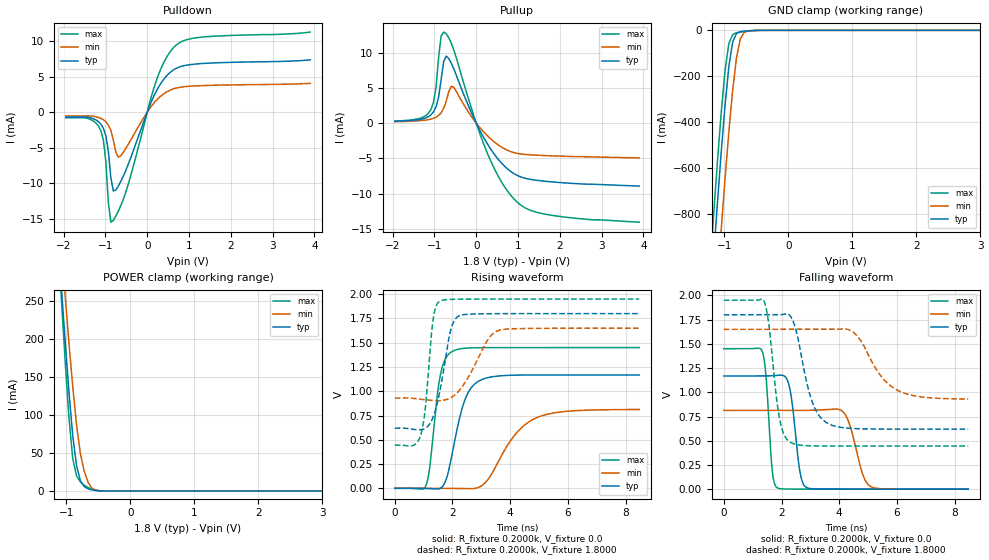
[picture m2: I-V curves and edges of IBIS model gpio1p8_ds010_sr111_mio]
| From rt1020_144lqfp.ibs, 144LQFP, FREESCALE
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[Model] gpio1p8_ds010_sr111_mio
|   Model gpio1p8_ds010_sr111_mio
| This model was characterised for following simulation conditions:
| External (pad) voltage:
|   - Typ: 1.8V,   - Min: 1.65V,   - Max: 1.95V
| Library cells for typ/min/max conditions are connected as defined below:
|  pad - External Pad
|  ipp_do - Core Input
|  ipp_obe - Output Buffer Enable
|  esd_boost - ovdd
|  ipp_dse0 - vssi
|  ipp_dse1 - vddi
|  ipp_dse2 - vssi
|  ipp_fsel0 - vddi
|  ipp_fsel1 - vddi
|  ipp_ina - ipp_ina
|  ipp_ind - ipp_ind
|  ipp_pwr_stable - vddi
|  ipp_sre - vddi
|  ovdd - ovdd
|  ovss - ovss
|  vddi - vddi
|  vssi - vssi
| All other pins connected to ground
Model_type I/O
Polarity   Non-Inverting
Enable   Active-High
Vinl =   0.5400V
Vinh =   1.2600V
Vmeas =  0.9000V
Cref =   0.0F
Rref =   0.2000k
Vref =   0.9000V
C_comp   1.2573pF   1.2208pF   1.3056pF
|C_comp_pullup   0.6440pF   0.6611pF   0.6285pF
|C_comp_pulldown   0.5474pF   0.5788pF   0.5258pF
[Model Spec]
| variable   typ   min   max
Vinh   1.2600V   1.1550V   1.3650V
Vinl   0.5400V   0.4950V   0.5850V
S_overshoot_high   1.8000V   1.6500V   1.9500V
S_overshoot_low   0.0V   0.0V   0.0V
Vmeas   0.9000V   0.8250V   0.9750V
Vref   0.9000V   0.8250V   0.9750V
Cref   0.0F   0.0F   0.0F
Rref   0.2000k   0.2000k   0.2000k
[Temperature Range]   25.0000   0.1050k   -20.0000
[Voltage Range]   1.8000V   1.6500V   1.9500V
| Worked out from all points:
|   slope of the pulldown table from 0 to 0.27 V, typ, clamps not added: 76.7 ohm
|   slope of the pullup table from 0 to 0.27 V, typ, clamps not added: 91 ohm
|   GND clamp passes 1 mA (typ) near -0.55 V on its own axis
|   POWER clamp passes 1 mA (typ) near -0.58 V on its own axis
|   rising waveform, R_fixture 0.2000k, V_fixture 0.0: 20-80 % time 556ps typ, 1.1ns min, 334ps max; typ from 0 V to 1.17 V
|   rising waveform, R_fixture 0.2000k, V_fixture 1.8000: 20-80 % time 431ps typ, 774ps min, 263ps max; typ from 0.619 V to 1.8 V
|   falling waveform, R_fixture 0.2000k, V_fixture 0.0: 20-80 % time 263ps typ, 424ps min, 185ps max; typ from 1.17 V to 0 V
|   falling waveform, R_fixture 0.2000k, V_fixture 1.8000: 20-80 % time 560ps typ, 950ps min, 339ps max; typ from 1.8 V to 0.619 V
[Pulldown]
|Voltage   I(typ)   I(min)   I(max)
-1.95V    -679uA     -527uA     -778uA
-1.41V    -700uA     -513uA     -902uA
-1.11V    -1.667mA   -870uA     -2.597mA
-990mV    -3.318mA   -1.338mA   -6.94mA
-930mV    -5.527mA   -1.788mA   -12.74mA
-870mV    -9.21mA    -2.57mA    -15.45mA
-810mV    -11.08mA   -3.94mA    -15.19mA
-750mV    -10.91mA   -5.632mA   -14.56mA
-630mV    -9.694mA   -6.09mA    -13.08mA
210mV     2.875mA    1.617mA    4.3mA
690mV     6.147mA    3.383mA    9.407mA
3.9V      7.35mA     4.05mA     11.25mA
[Pullup]
|Voltage   I(typ)   I(min)   I(max)
-1.95V    260uA      200uA      280uA
-1.08V    1.195mA    574uA      1.984mA
-960mV    2.342mA    845uA      5.218mA
-900mV    3.721mA    1.088mA    9.383mA
-840mV    6.196mA    1.468mA    12.37mA
-780mV    8.726mA    2.089mA    12.91mA
-720mV    9.498mA    3.099mA    12.69mA
-540mV    7.732mA    5.075mA    10.42mA
240mV     -2.675mA   -1.638mA   -3.883mA
960mV     -7.353mA   -4.267mA   -11.09mA
1.74V     -8.3mA     -4.625mA   -13.01mA
3.9V      -8.929mA   -4.938mA   -14.05mA
[GND_clamp]
|Voltage   I(typ)   I(min)   I(max)
-1.95V    -4.191A    -4.477A    -4.042A
-1.23V    -1.234A    -1.577A    -1.052A
-1.17V    -993.2mA   -1.338A    -811.1mA
-1.11V    -758.1mA   -1.102A    -578.5mA
-1.05V    -533.7mA   -870.8mA   -361.6mA
-990mV    -328mA     -648.8mA   -176.9mA
-930mV    -157.5mA   -441.8mA   -57.56mA
-870mV    -50.13mA   -259.5mA   -18.17mA
-810mV    -13.28mA   -118mA     -10.41mA
-750mV    -5.921mA   -36.52mA   -7.502mA
-630mV    -2.275mA   -2.653mA   -3.283mA
3.9V      0A         0A         0A
[POWER_clamp]
|Voltage   I(typ)   I(min)   I(max)
-1.95V    1.356A     1.328A     1.514A
-1.08V    270.6mA    322.7mA    256.8mA
-1.02V    199mA      258.1mA    173mA
-960mV    131.2mA    195.7mA    97.36mA
-900mV    72.67mA    137.2mA    42.48mA
-840mV    32.99mA    86.34mA    19.5mA
-780mV    13.32mA    48.87mA    11.87mA
-720mV    5.671mA    25.66mA    7.515mA
-660mV    2.793mA    11.19mA    4.477mA
-600mV    1.289mA    3.449mA    2.334mA
-480mV    122.1uA    182.3uA    260.9uA
3.9V      0A         0A         0A
[Ramp]
| variable   typ   min   max
dV/dt_r  0.7010/0.5561n   0.4872/1.1009n   0.8699/0.3344n
dV/dt_f  0.7084/0.5600n   0.4317/0.9504n   0.9030/0.3385n
R_load = 0.2000k
[Rising Waveform]
R_fixture= 0.2000k
V_fixture= 0.0
V_fixture_min= 0.0
V_fixture_max= 0.0
|time   V(typ)   V(min)   V(max)
0s        1.069nV    10.06nV    2.165nV
1.087ns   -2.116mV   168.2uV    32.82mV
1.218ns   -3.762mV   137.9uV    229.9mV
1.571ns   -1.592mV   -264.3uV   1.155V
1.971ns   330.3mV    -1.77mV    1.407V
2.412ns   897.3mV    -4.184mV   1.443V
2.988ns   1.117V     22.27mV    1.449V
4.08ns    1.165V     518.6mV    1.45V
4.794ns   1.168V     710.2mV    1.45V
8.47ns    1.168V     812mV      1.45V
[Rising Waveform]
R_fixture= 0.2000k
V_fixture= 1.8000
V_fixture_min= 1.6500
V_fixture_max= 1.9500
|time   V(typ)   V(min)   V(max)
0s        619.3mV    928.9mV    445mV
665.5ps   606mV      925.7mV    444.9mV
918ps     604.3mV    916.6mV    567.4mV
1.05ns    617.3mV    912.4mV    802.5mV
1.332ns   736mV      904.9mV    1.748V
1.551ns   981.4mV    903.5mV    1.926V
1.929ns   1.62V      930.7mV    1.947V
2.261ns   1.781V     1.017V     1.949V
3.623ns   1.8V       1.629V     1.95V
8.47ns    1.8V       1.65V      1.95V
[Falling Waveform]
R_fixture= 0.2000k
V_fixture= 0.0
V_fixture_min= 0.0
V_fixture_max= 0.0
|time   V(typ)   V(min)   V(max)
0s        1.168V     812.6mV    1.45V
1.339ns   1.168V     812.4mV    1.418V
1.688ns   1.171V     812.4mV    169.4mV
1.856ns   1.175V     812.4mV    13.21mV
2.274ns   1.058V     812.4mV    1.106mV
2.634ns   187.4mV    812.7mV    409.6uV
2.869ns   17.03mV    813.4mV    250.6uV
4.179ns   244.9uV    782.7mV    44.33uV
5.102ns   70.83uV    25.24mV    13.96uV
8.47ns    2.223uV    36.62uV    331.1nV
[Falling Waveform]
R_fixture= 0.2000k
V_fixture= 1.8000
V_fixture_min= 1.6500
V_fixture_max= 1.9500
|time   V(typ)   V(min)   V(max)
0s        1.8V       1.65V      1.95V
1.4ns     1.8V       1.65V      1.937V
1.564ns   1.8V       1.65V      1.695V
1.927ns   1.8V       1.65V      736.8mV
2.308ns   1.786V     1.65V      483.9mV
3.063ns   902.5mV    1.65V      447.1mV
3.588ns   681.2mV    1.65V      445.4mV
4.497ns   625.7mV    1.618V     445.1mV
6.015ns   619.4mV    1.022V     445mV
8.47ns    619.3mV    930.5mV    445mV
